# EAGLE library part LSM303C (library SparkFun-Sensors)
Ultra-compact high-performance eCompass module 3D accelerometer and 3D magnetometer Datasheet SparkFun Products SparkFun 6 Degrees of Freedom Breakout - LSM303C (BOB-13303)
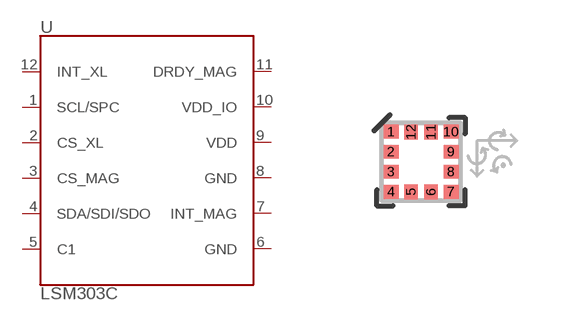
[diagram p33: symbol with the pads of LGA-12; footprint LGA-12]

Designator prefix U

## LSM303C (PROD_ID: IC-12557; VALUE: LSM303C)  [LGA-12]
1  SCL/SPC
2  CS_XL
3  CS_MAG
4  SDA/SDI/SDO
5  C1
6  GND
7  INT_MAG
8  GND
9  VDD
10  VDD_IO
11  DRDY_MAG
12  INT_XL

## Footprint LGA-12 (pad centres in mm)
LGA-12 2x2x1 mm 12-lead 0.50mm pitch Pads are 0.25x0.275 mm Derrived from the following ST PDFs http://www.st.com/st-web-ui/static/active/en/resource/technical/document/datasheet/DM00089896.pdf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
smd 0.375 x 0.35: 1 -0.75,0.75; 2 -0.75,0.25; 3 -0.75,-0.25; 4 -0.75,-0.75; 7 0.75,-0.75; 8 0.75,-0.25; 9 0.75,0.25; 10 0.75,0.75
smd 0.35 x 0.375: 5 -0.25,-0.75; 6 0.25,-0.75; 11 0.25,0.75; 12 -0.25,0.75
